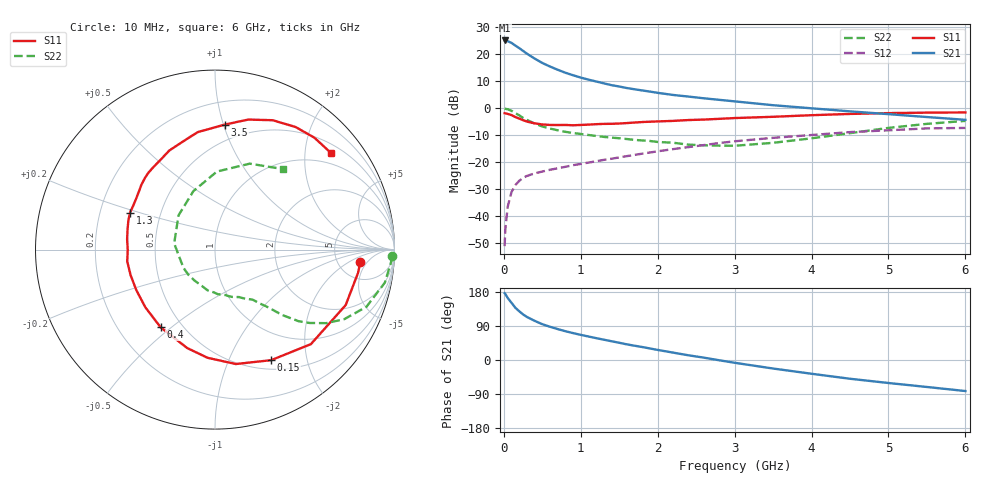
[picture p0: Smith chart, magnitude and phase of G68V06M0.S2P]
! SIEMENS Small Signal Semiconductors
! BFG193
! Si NPN RF Bipolar Junction Transistor in SOT223
! VCE = 8 V  IC = 6 mA
! Common Emitter S-Parameters:  August  1996
# GHz  S  MA  R  50
!  f  S11  S21  S12  S22
! GHz  MAG  ANG  MAG  ANG  MAG  ANG  MAG  ANG
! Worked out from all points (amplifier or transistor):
!   36 points, 10 MHz to 6 GHz, reference 50 ohm
!   highest |S21| = 25.2 dB at 10 MHz (marker M1)
!   |S21| within 3 dB of that: start of sweep to 207.8 MHz
!   unconditionally stable (mu >= 1): 1.082 GHz to 2.525 GHz
!   at 250 MHz: K = 0.38, MSG = 23.5 dB, |S12| = -25.8 dB
!   at 1.4 GHz: K = 1.08, MAG = 11.9 dB, |S12| = -18.7 dB
!   at 6 GHz: K = 0.86, MSG = 1.5 dB, |S12| = -7.2 dB
!   S11 on the Smith chart (normalised r, x): 10 MHz: 8.39, -3.30; 150 MHz: 0.61, -1.45; 400 MHz: 0.38, -0.46; 1.3 GHz: 0.33, +0.19; 3.5 GHz: 0.37, +1.01; 6 GHz: 0.71, +2.60
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0.01  0.8132 -4.7  18.13 176.4  0.0028 90.5  0.989 -2.2
0.02  0.8073 -9.3  18.02 174.1  0.0059 82.8  0.9824 -4.4
0.05  0.791 -23.0  17.59 163.7  0.015 77.7  0.9641 -11.0
0.1  0.7503 -44.6  16.33 150.9  0.0283 68.7  0.9018 -20.7
0.15  0.6908 -63.1  14.56 137.8  0.038 60.2  0.8177 -28.3
0.2  0.648 -79.7  13.08 128.6  0.0455 55.5  0.7426 -33.5
0.25  0.6043 -93.9  11.61 120.2  0.0515 50.7  0.6669 -37.8
0.3  0.5699 -105.8  10.32 113.6  0.056 47.9  0.613 -40.6
0.4  0.5284 -125.0  8.372 103.4  0.0626 44.5  0.5229 -44.2
0.5  0.5039 -140.4  6.94 94.5  0.0675 42.5  0.4627 -46.3
0.6  0.4931 -152.7  5.959 87.7  0.0729 42.2  0.423 -48.1
0.7  0.4914 -163.2  5.198 81.6  0.0776 42.4  0.393 -50.1
0.9  0.4862 -179.8  4.108 71.0  0.0887 42.6  0.3499 -53.0
1.1  0.5001 166.9  3.406 62.0  0.099 42.8  0.3214 -58.3
1.3  0.516 156.5  2.909 53.6  0.1112 42.7  0.2963 -63.2
1.6  0.5346 142.2  2.379 41.2  0.1305 40.9  0.2705 -73.6
2.2  0.5866 120.7  1.774 19.5  0.1759 34.8  0.231 -100.1
2.8  0.6403 103.1  1.44 -0.7  0.2279 25.1  0.2041 -136.8
3.5  0.6986 85.5  1.145 -22.5  0.2847 10.3  0.2301 171.4
4.5  0.7891 66.0  0.881 -49.5  0.3636 -9.9  0.3476 110.2
5.5  0.8339 48.4  0.691 -71.2  0.4259 -35.6  0.5165 68.0
6  0.8412 39.7  0.614 -81.9  0.4345 -50.3  0.5868 49.9
